|   Package Model For RM44xPGE
[IBIS Ver]   4.1
[File Name]   rm44x_pge.ibs
[File Rev]   1.0
[Date]   Thu Sep 4 18:41:18 2014
[Source]   Texas Instruments, Inc.
[Notes]   Revision History:
   1.0: initial release, 09/04/2014
   THIS IS RELEASE 1.0,THE CONTENTS ARE SUBJECT TO
   CHANGE WITHOUT PRIOR NOTICE,IF NECESSARY.
[Disclaimer] Please be aware that in the absence of a written agreement
   Texas Instruments(TI) assumes no liability for:
   (1) The accuracy of the IBIS models provided to your company
   (2) The proper functioning of these Models in your design
   or for any resulting applications;or
   (3) Infringement of patents,copyrights or intellectual
   property rights resulting from your use of these models.
   TI provides IBIS Models as a service to our customers and
   therefore reserves the right to limit distribution of the
   Models.
[Copyright]   Property of Texas Instruments Incorporated.
   Unauthorised reproduction and/or distribution is strictly.
   prohibited.
   This product is protected under copyright law and trade
   secret law as an unpublished work.
   Created 2013,(C) Copyright 2013-2014,
   Texas Instruments Incorporated., All Rights Reserved.
   These commodities are under the U.S. Government
   distribution license control.As such,they are not to be
   re-exported without the prior approval of the
   U.S. Department of Commerce.
[Component]   RM44xPGE
[Manufacturer]   Texas Instruments
[Package]
| variable   typ   min   max
R_pkg   303.058m   154.742m   347.374m
L_pkg   7.99408nH   5.8078nH   9.95738nH
C_pkg   0.647398pF   0.539097pF   0.817881pF
[Pin]   signal_name   model_name   R_pin   L_pin   C_pin
1	GIOB[3]	BQ0210FS_PD_3X2	323.014m	9.56542nH	0.64284pF
2	GIOA[0]	BQ0210FS_PD_3X2	319.428m	9.20674nH	0.775273pF
3	MIBSPI3NCS[3]	BQ0210FS_PU_3X2	316.029m	8.95547nH	0.748895pF
4	MIBSPI3NCS[2]	BQ0210FS_PU_3X2	312.388m	8.6955nH	0.713809pF
5	GIOA[1]	BQ0210FS_PD_3X2	310.29m	8.60899nH	0.695483pF
6	NHET1[11]	BQ0215FS_PD_3X2	307.207m	8.38798nH	0.672771pF
|7	FLTP1	TP1_220UM	303.073m	8.24237nH	0.635392pF
|8	FLTP2	BAFTHRU8VFT	304.617m	8.19212nH	0.61685pF
9	GIOA[2]	BQ0215FS_PD_3X2	315.066m	8.38527nH	0.609874pF
|10	VCCIO	0	208.821m	7.51139nH	0.681533pF
|11	VSS	0	320.966m	8.34366nH	0.635075pF
12	CAN3RX	BQ0210FS_PU_3X2	319.843m	8.25447nH	0.608887pF
13	CAN3TX	BQ0210FS_PU_3X2	324.78m	8.33552nH	0.58501pF
14	GIOA[5]	BQ0215FS_PD_3X2	327.995m	8.38026nH	0.609739pF
15	NHET1[22]	BQ0215FS_PD_3X2	330.139m	8.23609nH	0.621577pF
16	GIOA[6]	BQ0215FS_PD_3X2	333.148m	8.14031nH	0.617585pF
|17	VCC	0	174.492m	6.6831nH	0.722325pF
|18	OSCIN	0	332.846m	8.19616nH	0.57845pF
|19	KELVIN_GND	0	335.23m	8.19846nH	0.593462pF
|20	OSCOUT	0	333.22m	8.15861nH	0.602437pF
|21	VSS	0	214.109m	7.06008nH	0.673082pF
22	GIOA[7]	BQ0215FS_PD_3X2	324.083m	8.00494nH	0.604611pF
23	NHET1[01]	BQ0215FS_PD_3X2	323.243m	7.99573nH	0.616688pF
24	NHET1[03]	BQ0215FS_PD_3X2	322.947m	8.03225nH	0.622391pF
25	NHET1[0]	BQ0215FS_PD_3X2	322.149m	8.03538nH	0.630137pF
|26	VCCIO	0	219.282m	7.07691nH	0.723849pF
|27	VSS	0	332.218m	7.98477nH	0.649857pF
|28	VSS	0	331.818m	8.06339nH	0.660009pF
|29	VCC	0	181.333m	6.68073nH	0.817881pF
30	NHET1[02]	BQ0215FS_PD_3X2	331.001m	8.24631nH	0.689593pF
31	NHET1[05]	BQ0215FS_PD_3X2	331.527m	8.44197nH	0.68672pF
32	MIBSPI5NCS[0]	BQ0215FS_PU_3X2	331.005m	8.50365nH	0.70434pF
33	NHET1[07]	BQ0215FS_PD_3X2	336.049m	8.66715nH	0.736296pF
34	TEST	BQ0213FS_PD_3X2	337.905m	8.89321nH	0.760931pF
35	NHET1[09]	BQ0215FS_PD_3X2	342.568m	9.16817nH	0.784717pF
36	NHET1[04]	BQ0215FS_PD_3X2	347.374m	9.57074nH	0.646239pF
37	MIBSPI3NCS[1]	BQ0215FS_PU_3X2	316.195m	9.31645nH	0.63734pF
38	NHET1[06]	BQ0215FS_PD_3X2	308.741m	8.85838nH	0.760439pF
39	NHET1[13]	BQ0215FS_PD_3X2	304.655m	8.60826nH	0.737796pF
40	MIBSPI1NCS[2]	BQ0215FS_PU_3X2	298.423m	8.36279nH	0.722066pF
41	NHET1[15]	BQ0215FS_PD_3X2	292.471m	8.12966nH	0.698104pF
|42	VCCIO	0	289.765m	7.91884nH	0.674838pF
|43	VSS	0	286.737m	7.7006nH	0.653722pF
|44	VSS	0	285.479m	7.50301nH	0.639247pF
|45	VCC	0	154.742m	6.34786nH	0.7375pF
46	nPORRST	IQ0087FS_3X2	289.825m	7.42311nH	0.613803pF
|47	VSS	0	287.754m	7.2699nH	0.604318pF
|48	VCC	0	191.583m	6.32645nH	0.674007pF
|49	VCC	0	192.637m	6.30214nH	0.660978pF
|50	VSS	0	291.149m	7.09233nH	0.567684pF
51	MIBSPI3SOMI	BT3304BHYPU_AICLN_3X2SF	291.14m	7.11473nH	0.544072pF
52	MIBSPI3SIMO	BT3304BHYPU_AICLN_3X2SF	291.326m	7.14696nH	0.549958pF
53	MIBSPI3CLK	BT3304BHYPU_AICLN_3X2SF	292.853m	7.10587nH	0.558284pF
54	MIBSPI3NENA	BQ0210FS_PU_3X2	298.412m	7.10002nH	0.559032pF
55	MIBSPI3NCS[0]	BQ0215FS_PU_3X2	303.029m	7.20567nH	0.550184pF
|56	VSS	0	299.499m	7.18187nH	0.552479pF
|57	VCC	0	299.255m	7.25977nH	0.545088pF
|58	AD1IN[16]_AD2IN[0]	ARCHER_ADC	286.961m	7.02759nH	0.540093pF
|59	AD1IN[17]_AD2IN[01]	ARCHER_ADC	290.696m	7.03291nH	0.570677pF
|60	AD1IN[0]	ARCHER_ADC	290.186m	7.09816nH	0.586428pF
|61	AD1IN[07]	ARCHER_ADC	293.188m	7.23291nH	0.597903pF
|62	AD1IN[18]_AD2IN[02]	ARCHER_ADC	293.732m	7.39748nH	0.608103pF
|63	AD1IN[19]_AD2IN[03]	ARCHER_ADC	295.864m	7.52284nH	0.620657pF
|64	AD1IN[20]_AD2IN[04]	ARCHER_ADC	305.587m	7.68076nH	0.634287pF
|65	AD1IN[21]_AD2IN[05]	ARCHER_ADC	313.968m	7.79583nH	0.636484pF
|66	ADREFHI	ARCHER_ADC	310.896m	7.87639nH	0.641105pF
|67	ADREFLO	0	314.118m	8.01409nH	0.669125pF
|68	VSSAD	0	317.478m	8.15156nH	0.696795pF
|69	VCCAD	ARCHER_ADC	323.404m	8.41656nH	0.72474pF
|70	AD1IN[09]_AD2IN[09]	ARCHER_ADC	329.723m	8.75531nH	0.759691pF
|71	AD1IN[01]	ARCHER_ADC	336.092m	9.1767nH	0.794177pF
|72	AD1IN[10]_AD2IN[10]	ARCHER_ADC	344.701m	9.57073nH	0.666989pF
|73	AD1IN[02]	ARCHER_ADC	341.237m	9.95738nH	0.679816pF
|74	AD1IN[03]	ARCHER_ADC	330.567m	9.34754nH	0.805819pF
|75	AD1IN[11]_AD2IN[11]	ARCHER_ADC	316.118m	8.9683nH	0.740881pF
|76	AD1IN[04]	ARCHER_ADC	299.871m	8.44072nH	0.692286pF
|77	AD1IN[12]_AD2IN[12]	ARCHER_ADC	299.454m	8.28105nH	0.690868pF
|78	AD1IN[05]	ARCHER_ADC	298.175m	8.15506nH	0.677186pF
|79	AD1IN[13]_AD2IN[13]	ARCHER_ADC	299.279m	8.10844nH	0.663778pF
|80	AD1IN[06]	ARCHER_ADC	298.435m	8.02054nH	0.651581pF
|81	AD1IN[22]_AD2IN[06]	ARCHER_ADC	302.953m	7.97121nH	0.640861pF
|82	AD1IN[14]_AD2IN[14]	ARCHER_ADC	305.88m	7.93257nH	0.631694pF
|83	AD1IN[08]_AD2IN[08]	ARCHER_ADC	307.539m	7.84754nH	0.625176pF
|84	AD1IN[23]_AD2IN[07]	ARCHER_ADC	310.742m	7.81609nH	0.619299pF
|85	AD1IN[15]_AD2IN[15]	ARCHER_ADC	318.664m	7.89458nH	0.592529pF
86	AD1EVT	BQ0210FS_PD_3X2	324.388m	8.0116nH	0.562049pF
|87	VCC	0	173.165m	6.53287nH	0.706306pF
|88	VSS	0	329.16m	8.03606nH	0.611662pF
89	CAN1TX	BQ0210FS_PU_3X2	336.721m	8.04162nH	0.606408pF
90	CAN1RX	BQ0210FS_PU_3X2	338.914m	8.10755nH	0.602516pF
91	NHET1[24]	BQ0210FS_PD_3X2	334.621m	8.24269nH	0.585955pF
92	NHET1[26]	BQ0210FS_PD_3X2	333.649m	8.21313nH	0.589638pF
93	MIBSPI1SIMO	BT3304BHYPU_AICLN_3X2SF	332.884m	8.32073nH	0.612345pF
94	MIBSPI1SOMI	BT3304BHYPU_AICLN_3X2SF	331.808m	8.34231nH	0.600523pF
95	MIBSPI1CLK	BT3304BHYPU_AICLN_3X2SF	332.519m	8.26129nH	0.60207pF
96	MIBSPI1NENA	BQ0215FS_PU_3X2	337.437m	8.37904nH	0.609072pF
97	MIBSPI5NENA	BQ0215FS_PU_3X2	330.254m	8.32955nH	0.591293pF
98	MIBSPI5SOMI[0]	BT3308BHYPP_AIC_3X2SF	330.781m	8.25946nH	0.601889pF
99	MIBSPI5SIMO[0]	BT3308BHYPP_AIC_3X2SF	331.352m	8.20279nH	0.631286pF
100	MIBSPI5CLK	BT3308BHYPP_AIC_3X2SF	328.82m	8.35817nH	0.642112pF
|101	VCC	0	213.786m	7.33715nH	0.705421pF
|102	VSS	0	324.395m	8.3392nH	0.661504pF
|103	VSS	0	325.797m	8.42097nH	0.671628pF
|104	VCCIO	0	327.641m	8.55922nH	0.704208pF
105	MIBSPI1NCS[0]	BQ0215FS_PU_3X2	331.257m	8.79797nH	0.737128pF
106	NHET1[08]	BQ0215FS_PD_3X2	331.985m	9.0053nH	0.763792pF
107	NHET1[28]	BQ0215FS_PD_3X2	339.882m	9.27582nH	0.784746pF
108	TMS	BT3308BHYPP_AIC_3X2SF	345.272m	9.62684nH	0.644594pF
109	nTRST	IQ0087FS_3X2	319.874m	9.54667nH	0.63989pF
110	TDI	BQ0192FS_PU_3X2	314.176m	9.16171nH	0.777303pF
111	TDO	BT3308BHYPP_AIC_3X2SF	307.03m	8.83785nH	0.752427pF
112	TCK	IQ0079FS_PD_3X2	301.912m	8.61018nH	0.724882pF
113	RTCK	BT3308BHYPP_AIC_3X2SF	296.973m	8.32441nH	0.684643pF
|114	VCC	0	298.36m	8.26193nH	0.669136pF
|115	VSS	0	294.2m	8.03594nH	0.665341pF
116	nRST	BT3304BHYPD_AICDL_3X2SF	291.415m	7.87815nH	0.645803pF
117	nERROR	BT3308BHYPP_AIC_3X2SF	292.115m	7.69942nH	0.629928pF
118	NHET1[10]	BQ0215FS_PD_3X2	287.643m	7.57059nH	0.615049pF
119	ECLK	BQ0215FS_PD_3X2	288.622m	7.45986nH	0.602583pF
|120	VCCIO	0	284.492m	7.38404nH	0.591566pF
|121	VSS	0	287.439m	7.31955nH	0.581808pF
|122	VSS	0	289.529m	7.24509nH	0.57266pF
|123	VCC	0	291m	7.25132nH	0.566068pF
124	NHET1[12]	BQ0210FS_PD_3X2	293.169m	7.20438nH	0.560749pF
125	NHET1[14]	BQ0215FS_PD_3X2	293.987m	7.23683nH	0.54636pF
126	GIOB[0]	BQ0215FS_PD_3X2	298.806m	7.28398nH	0.543158pF
127	NHET1[30]	BQ0215FS_PD_3X2	297.797m	7.17431nH	0.553063pF
128	CAN2TX	BQ0210FS_PU_3X2	298.664m	7.14815nH	0.539101pF
129	CAN2RX	BQ0210FS_PU_3X2	295.573m	7.09409nH	0.539097pF
130	MIBSPI1NCS[1]	BQ0215FS_PU_3X2	295.025m	7.18135nH	0.557611pF
131	LINRX	BQ0210FS_PU_3X2	296.312m	7.13965nH	0.565786pF
132	LINTX	BQ0210FS_PU_3X2	296.701m	7.25502nH	0.585218pF
133	GIOB[1]	BQ0215FS_PD_3X2	300.78m	7.31137nH	0.586654pF
|134	VCCP	0	166.717m	5.8078nH	0.725192pF
|135	VSS	0	296.895m	7.24526nH	0.595356pF
|136	VCCIO	0	289.725m	7.30759nH	0.600681pF
|137	VCC	0	292.399m	7.43303nH	0.62851pF
|138	VSS	0	295.422m	7.56134nH	0.647001pF
139	NHET1[16]	BQ0215FS_PD_3X2	300.673m	7.74213nH	0.667934pF
140	NHET1[18]	BQ0215FS_PD_3X2	305.422m	7.91715nH	0.690547pF
141	NHET1[20]	BQ0215FS_PD_3X2	312.05m	8.16752nH	0.714152pF
142	GIOB[2]	BQ0210FS_PD_3X2	319.936m	8.467nH	0.741146pF
|143	VCC	0	326.905m	8.79539nH	0.771122pF
|144	VSS	0	333.697m	9.2177nH	0.645112pF
[Model Selector] BQ0192FS_PU_3X2
BQ0192FS_PU_3X2_PZ_3P3  Cell operated at 3.3(nom)
|BQ0192FS_PU_3X2_PZ_3P3; PUPD_OFF
BQ0192FS_PU_3X2_PU_3P3  Cell operated at 3.3(nom)
|BQ0192FS_PU_3X2_PU_3P3; PULLUP_ON
BQ0192FS_PU_3X2_PD_3P3  Cell operated at 3.3(nom)
|BQ0192FS_PU_3X2_PD_3P3; PULLDOWN_ON
[Model Selector] BQ0210FS_PU_3X2
BQ0210FS_PU_3X2_PZ_3P3  Cell operated at 3.3(nom)
|BQ0210FS_PU_3X2_PZ_3P3; PUPD_OFF
BQ0210FS_PU_3X2_PU_3P3  Cell operated at 3.3(nom)
|BQ0210FS_PU_3X2_PU_3P3; PULLUP_ON
BQ0210FS_PU_3X2_PD_3P3  Cell operated at 3.3(nom)
|BQ0210FS_PU_3X2_PD_3P3; PULLDOWN_ON
[Model Selector] BQ0210FS_PD_3X2
BQ0210FS_PD_3X2_PZ_3P3  Cell operated at 3.3(nom)
|BQ0210FS_PD_3X2_PZ_3P3; PUPD_OFF
BQ0210FS_PD_3X2_PU_3P3  Cell operated at 3.3(nom)
|BQ0210FS_PD_3X2_PU_3P3; PULLUP_ON
BQ0210FS_PD_3X2_PD_3P3  Cell operated at 3.3(nom)
|BQ0210FS_PD_3X2_PD_3P3; PULLDOWN_ON
[Model Selector] BQ0213FS_PD_3X2
BQ0213FS_PD_3X2_PD_3P3  Cell operated at 3.3(nom)
|BQ0213FS_PD_3X2_PD_3P3; PULLDOWN_ON
BQ0213FS_PD_3X2_PZ_3P3  Cell operated at 3.3(nom)
|BQ0213FS_PD_3X2_PZ_3P3; PULLUP_OFF
[Model Selector] BQ0215FS_PD_3X2
BQ0215FS_PD_3X2_PZ_3P3  Cell operated at 3.3(nom)
|BQ0215FS_PD_3X2_PZ_3P3; PUPD_OFF
BQ0215FS_PD_3X2_PU_3P3  Cell operated at 3.3(nom)
|BQ0215FS_PD_3X2_PU_3P3; PULLUP_ON
BQ0215FS_PD_3X2_PD_3P3  Cell operated at 3.3(nom)
|BQ0215FS_PD_3X2_PD_3P3; PULLDOWN_ON
[Model Selector] BQ0215FS_PU_3X2
BQ0215FS_PU_3X2_PZ_3P3  Cell operated at 3.3(nom)
|BQ0215FS_PU_3X2_PZ_3P3; PUPD_OFF
BQ0215FS_PU_3X2_PU_3P3  Cell operated at 3.3(nom)
|BQ0215FS_PU_3X2_PU_3P3; PULLUP_ON
BQ0215FS_PU_3X2_PD_3P3  Cell operated at 3.3(nom)
|BQ0215FS_PU_3X2_PD_3P3; PULLDOWN_ON
[Model Selector] BT3304BHYPD_AICDL_3X2SF
BT3304BHYPD_AICDL_3X2SF_PZ_3P3  Cell operated at 3.3(nom)
|BT3304BHYPD_AICDL_3X2SF_PZ_3P3; PUPD_OFF
BT3304BHYPD_AICDL_3X2SF_PU_3P3  Cell operated at 3.3(nom)
|BT3304BHYPD_AICDL_3X2SF_PU_3P3; PULLUP_ON
BT3304BHYPD_AICDL_3X2SF_PD_3P3  Cell operated at 3.3(nom)
|BT3304BHYPD_AICDL_3X2SF_PD_3P3; PULLDOWN_ON
[Model Selector] BT3304BHYPU_AICLN_3X2SF
BT3304BHYPU_AICLN_3X2SF_PZ_3P3  Cell operated at 3.3(nom)
|BT3304BHYPU_AICLN_3X2SF_PZ_3P3; PUPD_OFF
BT3304BHYPU_AICLN_3X2SF_PU_3P3  Cell operated at 3.3(nom)
|BT3304BHYPU_AICLN_3X2SF_PU_3P3; PULLUP_ON
BT3304BHYPU_AICLN_3X2SF_PD_3P3  Cell operated at 3.3(nom)
|BT3304BHYPU_AICLN_3X2SF_PD_3P3; PULLDOWN_ON
[Model Selector] BT3308BHYPP_AIC_3X2SF
BT3308BHYPP_AIC_3X2SF_PZ_3P3  Cell operated at 3.3(nom)
|BT3308BHYPP_AIC_3X2SF_PZ_3P3; PUPD_OFF
BT3308BHYPP_AIC_3X2SF_PU_3P3  Cell operated at 3.3(nom)
|BT3308BHYPP_AIC_3X2SF_PU_3P3; PULLUP_ON
BT3308BHYPP_AIC_3X2SF_PD_3P3  Cell operated at 3.3(nom)
|BT3308BHYPP_AIC_3X2SF_PD_3P3; PULLDOWN_ON
[Model Selector] IQ0079FS_PD_3X2
079FS_PD_3X2_3P3  Cell operated at 3.3(nom)
|IQ0079FS_PD_3X2_3P3; PUPD_OFF
FS_PD_3X2_PU_3P3  Cell operated at 3.3(nom)
|IQ0079FS_PD_3X2_PU_3P3; PULLUP_ON
FS_PD_3X2_PD_3P3  Cell operated at 3.3(nom)
|IQ0079FS_PD_3X2_PD_3P3; PULLDOWN_ON
[Model Selector] IQ0087FS_3X2
087FS_3X2_PD_3P3  Cell operated at 3.3(nom)
|IQ0087FS_3X2_PD_3P3; PULLDOWN_ON
IQ0087FS_3X2_3P3  Cell operated at 3.3(nom)
| Models and submodels in the file (31): BQ0192FS_PU_3X2_PZ_3P3 (I/O), BQ0192FS_PU_3X2_PU_3P3 (I/O), BQ0192FS_PU_3X2_PD_3P3 (I/O), BQ0210FS_PU_3X2_PZ_3P3 (I/O), BQ0210FS_PU_3X2_PU_3P3 (I/O), BQ0210FS_PU_3X2_PD_3P3 (I/O), BQ0210FS_PD_3X2_PZ_3P3 (I/O), BQ0210FS_PD_3X2_PU_3P3 (I/O), BQ0210FS_PD_3X2_PD_3P3 (I/O), BQ0213FS_PD_3X2_PD_3P3 (I/O), BQ0213FS_PD_3X2_PZ_3P3 (I/O), BQ0215FS_PD_3X2_PZ_3P3 (I/O), BQ0215FS_PD_3X2_PU_3P3 (I/O), BQ0215FS_PD_3X2_PD_3P3 (I/O), BQ0215FS_PU_3X2_PZ_3P3 (I/O), BQ0215FS_PU_3X2_PU_3P3 (I/O), BQ0215FS_PU_3X2_PD_3P3 (I/O), BT3304BHYPD_AICDL_3X2SF_PZ_3P3 (I/O), BT3304BHYPD_AICDL_3X2SF_PU_3P3 (I/O), BT3304BHYPD_AICDL_3X2SF_PD_3P3 (I/O), BT3304BHYPU_AICLN_3X2SF_PZ_3P3 (I/O), BT3304BHYPU_AICLN_3X2SF_PU_3P3 (I/O), BT3304BHYPU_AICLN_3X2SF_PD_3P3 (I/O), BT3308BHYPP_AIC_3X2SF_PZ_3P3 (I/O), BT3308BHYPP_AIC_3X2SF_PU_3P3 (I/O), BT3308BHYPP_AIC_3X2SF_PD_3P3 (I/O), 079FS_PD_3X2_3P3 (Input), FS_PD_3X2_PU_3P3 (Input), FS_PD_3X2_PD_3P3 (Input), 087FS_3X2_PD_3P3 (Input), IQ0087FS_3X2_3P3 (Input)
